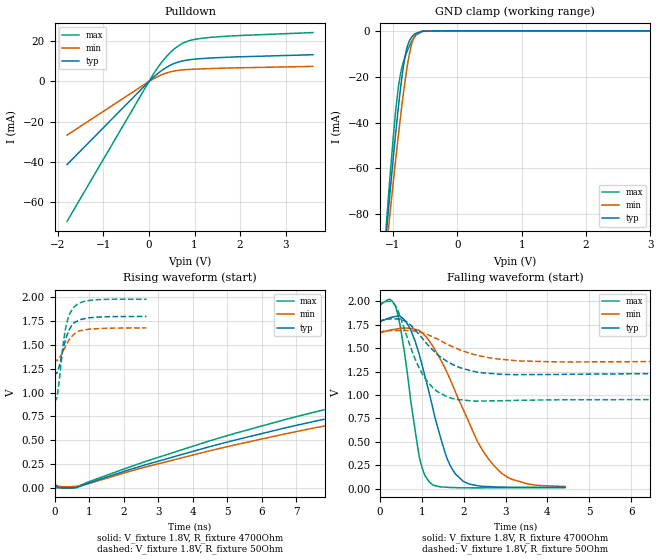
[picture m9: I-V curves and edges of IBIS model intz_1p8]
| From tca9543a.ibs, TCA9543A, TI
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|   intz_1p8 Model
[Model]   intz_1p8
Model_type   Open_drain
Polarity   Non-Inverting
Vmeas = 0.9
Vref = 1.8
Cref = 100pF
Rref = 4700
|   typ   min   max
|   (nom PVT)   (fast PVT)   (slow PVT)
C_comp   1.601e-12   1.523e-12   1.756e-12
| Where nom  PVT is Nominal Process, 1.8V, 27C
|   Fast PVT is Strong Process,  1.98V, -40C
|   Slow PVT is Weak Process,   1.68V, 85C
[Voltage Range]   1.8   1.68   1.98
|Junction Temperature
[Temperature Range]   27   85   -40
[Pullup Reference]   1.8   1.68   1.98
[Pulldown Reference]   0   0   0
[Power Clamp Reference]   1.8   1.68   1.98
[GND Clamp Reference]   0   0   0
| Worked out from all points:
|   slope of the pulldown table from 0 to 0.27 V, typ, clamps not added: 51.2 ohm
|   GND clamp passes 1 mA (typ) near -0.64 V on its own axis
|   falling waveform, V_fixture 1.8V, R_fixture 4700Ohm: 20-80 % time 632ps typ, 1.05ns min, 377ps max; typ from 1.8 V to 0.016 V
|   rising waveform, V_fixture 1.8V, R_fixture 4700Ohm: 20-80 % time 18.7ns typ, 19.6ns min, 17.8ns max; typ from 0.017 V to 1.8 V
|   falling waveform, V_fixture 1.8V, R_fixture 50Ohm: 20-80 % time 807ps typ, 1.04ns min, 581ps max; typ from 1.8 V to 1.23 V
|   rising waveform, V_fixture 1.8V, R_fixture 50Ohm: 20-80 % time 287ps typ, 342ps min, 242ps max; typ from 1.23 V to 1.8 V
[Pulldown]
|   Voltage   I(typ)   I(min)   I(max)
-1.8V     -41.18mA   -26.61mA   -69.32mA
90.9mV    1.966mA    1.226mA    3.412mA
203.4mV   4.136mA    2.548mA    7.225mA
358.2mV   6.624mA    3.994mA    11.71mA
581.9mV   9.158mA    5.287mA    16.61mA
713.3mV   10.06mA    5.655mA    18.6mA
855.2mV   10.65mA    5.901mA    20.01mA
1.113V    11.26mA    6.196mA    21.26mA
1.975V    12.2mA     6.758mA    22.74mA
3.6V      13.24mA    7.453mA    24.22mA
[GND Clamp]
|   Voltage   I(typ)   I(min)   I(max)
-1.8V     -330.7mA   -309.4mA   -374.5mA
-1.121V   -94.41mA   -100.9mA   -91.66mA
-1.084V   -82.63mA   -90.44mA   -77.7mA
-1.04V    -69.07mA   -78.31mA   -61.84mA
-976.3mV  -50.3mA    -61.35mA   -40.79mA
-926.8mV  -36.57mA   -48.65mA   -27.26mA
-883.3mV  -25.55mA   -38mA      -18.98mA
-835.7mV  -15.36mA   -27.16mA   -13.45mA
-775.8mV  -6.848mA   -15.27mA   -8.688mA
-714.7mV  -2.952mA   -6.418mA   -4.94mA
-637.4mV  -1.006mA   -1.314mA   -1.801mA
3.6V      0A         0A         0A
[POWER Clamp]
|   Voltage   I(typ)   I(min)   I(max)
-1.8V     0A         0A         0A
-1.706V   0A         0A         0A
3.6V      0A         0A         0A
[Ramp]
R_load = 4700
|   typ   min   max
dV/dt_r   1.06987/1.86261e-08   0.992949/1.95645e-08   1.18154/1.77349e-08
dV/dt_f   1.06987/6.31453e-10   0.992949/1.04841e-09   1.18154/3.76622e-10
[Falling Waveform]
V_fixture = 1.8V
V_fixture_min = 1.68V
V_fixture_max = 1.98V
R_fixture = 4700Ohm
|   Time   V(typ)   V(min)   V(max)
0s        1.8V       1.68V      1.98V
250ps     1.826V     1.694V     2.019V
410ps     1.843V     1.707V     1.885V
660ps     1.755V     1.714V     1.211V
930ps     1.445V     1.691V     359mV
1.18ns    1.015V     1.576V     70.9mV
1.61ns    313.4mV    1.233V     14.9mV
2ns       75.87mV    833.8mV    9.462mV
2.91ns    16.92mV    164.5mV    10.1mV
4.42ns    15.78mV    23.21mV    11.08mV
[Rising Waveform]
V_fixture = 1.8V
V_fixture_min = 1.68V
V_fixture_max = 1.98V
R_fixture = 4700Ohm
|   Time   V(typ)   V(min)   V(max)
0s        16.88mV    25.08mV    10.76mV
620ps     1.365mV    16.8mV     6.557mV
4.46ns    429.8mV    386.5mV    490.5mV
6.98ns    654.8mV    589.8mV    745.8mV
12.38ns   1.028V     930mV      1.164V
18.95ns   1.33V      1.21V      1.495V
26.6ns    1.544V     1.415V     1.726V
37.27ns   1.698V     1.569V     1.888V
47.16ns   1.763V     1.636V     1.951V
83.97ns   1.802V     1.681V     1.982V
[Falling Waveform]
V_fixture = 1.8V
V_fixture_min = 1.68V
V_fixture_max = 1.98V
R_fixture = 50Ohm
|   Time   V(typ)   V(min)   V(max)
0s        1.8V       1.68V      1.98V
250ps     1.813V     1.688V     2.002V
370ps     1.813V     1.688V     1.954V
660ps     1.774V     1.687V     1.603V
1.06ns    1.578V     1.658V     1.19V
1.35ns    1.442V     1.602V     1.044V
1.73ns    1.327V     1.517V     962mV
2.41ns    1.239V     1.415V     935.4mV
3.4ns     1.218V     1.363V     944.2mV
9.82ns    1.229V     1.36V      950.2mV
[Rising Waveform]
V_fixture = 1.8V
V_fixture_min = 1.68V
V_fixture_max = 1.98V
R_fixture = 50Ohm
|   Time   V(typ)   V(min)   V(max)
0s        1.228V     1.36V      950mV
40ps      1.202V     1.339V     928.2mV
80ps      1.22V      1.339V     989.2mV
250ps     1.463V     1.444V     1.53V
320ps     1.565V     1.493V     1.687V
420ps     1.661V     1.556V     1.818V
550ps     1.731V     1.611V     1.897V
720ps     1.764V     1.65V      1.943V
1.05ns    1.788V     1.669V     1.971V
2.66ns    1.8V       1.68V      1.98V
